(* Logix 5000 AddOnInstructionDefinition export YAI_Assy_72_73_115_EIP_Hz; software revision 21.03 *)

ADD_ON_INSTRUCTION YAI_Assy_72_73_115_EIP_Hz   (* revision 1.0, vendor Yaskawa America, Inc. *)
// YAI Assembly 72/73 and 115
// Help:
// This add-on instruction is for use with input assemblie 72/73 and output assemblies 115.
// Node_Input_Assy is defined as the node's input assembly integer array.
// Node_Output_Assy is defined as the node's output assembly integer array.
// Torque limit/reference, torque compensation and torque output variables are only available with A1000.
VAR_IN_OUT
   Node_Input_Assy : AB:ETHERNET_MODULE_INT_6Bytes:I:0; {required}   // Input assembly words
   Node_Output_Assy : AB:ETHERNET_MODULE_INT_40Bytes:O:0; {required}   // Output assembly words
END_VAR
VAR_INPUT
   RunFwd : BOOL; {visible}   // Forward run command
   RunRev : BOOL; {visible}   // Reverse run command
   MFI_3 : BOOL; {visible}   // Multi-function input 3
   MFI_4 : BOOL; {visible}   // Multi-function input 4
   MFI_5 : BOOL; {visible}   // Multi-function input 5
   MFI_6 : BOOL; {visible}   // Multi-function input 6
   MFI_7 : BOOL; {visible}   // Multi-function input 7
   MFI_8 : BOOL; {visible}   // Multi-function input 8
   External_Fault : BOOL;   // External fault command (EF0)
   FaultReset : BOOL; {visible}   // Fault reset command
   MFO_1 : BOOL; {visible}   // Multi-function output (M1-M2 for A/P1000, MA/MB/MC for V1000)
   MFO_2 : BOOL; {visible}   // Multi-function output (M3-M4 for A/P1000, P1 for V1000)
   MFO_3 : BOOL; {visible}   // Multi-function output (M5-M6 for A/P1000, P2 for V1000)
   Freq_Ref : REAL; {visible}   // Frequency reference command in Hz (xx.xx resolution)
   Torq_Ref_Limit : REAL; {visible}   // Torque reference/limit (A1000 only)
   Torq_Comp : REAL; {visible}   // Torque compensation command (A1000 only)
   Analog_Output_1 : REAL;   // Analog output 1 level command
   Analog_Output_2 : REAL;   // Analog output 2 level command
   Digital_Output_1 : BOOL;   // Digital output 1 activation - M1-M2
   Digital_Output_2 : BOOL;   // Digital output 2 activation - M3-M4
   Digital_Output_3 : BOOL;   // Digital output 3 activation - M5-M6
   Digital_Output_Fault_Enable : BOOL;   // Bit to enable control of fault output relay over the network
   Digital_Output_Fault : BOOL;   // Fault relay activation - MA-MB-MC
END_VAR
VAR_OUTPUT
   At_Speed : BOOL; {access Read Only, visible}   // Drive at commanded speed status bit
   Drive_State : INT; {access Read Only}   // Drive Status - Refer to class 0x29, Instance 0x1, Attribute 0x6 for details
   Faulted : BOOL; {access Read Only, visible}   // Drive faulted status bit
   NetCtrlStatus : BOOL; {access Read Only, visible}   // Drive network run source status bit (1 = source coming from network)
   NetRefStatus : BOOL; {access Read Only, visible}   // Drive network reference status bit (1 = reference coming from network)
   Output_Freq : REAL; {access Read Only, visible}   // Drive output frequency in Hz (xx.xx resolution)
   Ready : BOOL; {access Read Only, visible}   // Drive ready status bit
   RunningFwd : BOOL; {access Read Only, visible}   // Drive running forward status bit
   RunningRev : BOOL; {access Read Only, visible}   // Drive running reverse status bit
   Torque_Actual : REAL; {access Read Only, visible}   // Drive torque output in engineering units.
   Warning : BOOL; {access Read Only, visible}   // Drive warning (alarm) status bit
END_VAR
VAR_INPUT
   Motor_Rated_Torq : REAL := 100.0; {visible}   // Motor rated torque (Engineering units)
END_VAR
VAR
   FRef_Convert : DINT;
   FOut_Convert : REAL;
   FOut_Temp : REAL;
   TRef_Convert : INT;
   TComp_Convert : INT;
   TOut_Convert : REAL;
   TOut_Temp : REAL;
   IOut_Temp : REAL;
   IOut_Convert : REAL;
   AO1_Convert : INT;
   AO2_Convert : INT;
   Motor_Speed_Temp : REAL;
   Motor_Speed_Convert : REAL;
   Freq_Cmd_Temp : REAL;
   Freq_Cmd_Convert : REAL;
   AI1_Temp : REAL;
   AI1_Convert : REAL;
   AI2_Temp : REAL; {access None}
   AI2_Convert : REAL; {access None}
   AI3_Temp : REAL; {access None}
   AI3_Convert : REAL; {access None}
   TOut_Convert1 : REAL;
   Tout_Convert_Temp : REAL;
   TOut_Temp1 : REAL;
   TRef_Convert1 : INT;
   DriveStatusTempBits : INT;
END_VAR

ROUTINE Logic   (* ladder *)
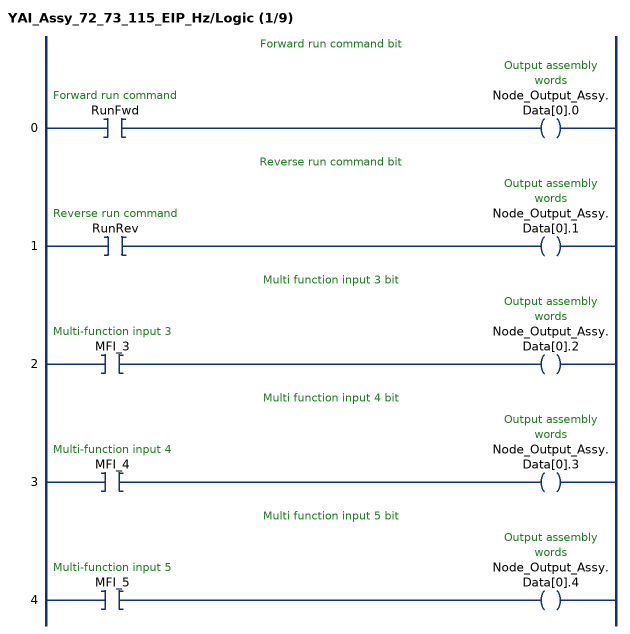
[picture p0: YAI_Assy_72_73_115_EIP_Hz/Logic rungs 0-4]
   // Forward run command bit
   0: XIC(RunFwd)OTE(Node_Output_Assy.Data[0].0);
   // Reverse run command bit
   1: XIC(RunRev)OTE(Node_Output_Assy.Data[0].1);
   // Multi function input 3 bit
   2: XIC(MFI_3)OTE(Node_Output_Assy.Data[0].2);
   // Multi function input 4 bit
   3: XIC(MFI_4)OTE(Node_Output_Assy.Data[0].3);
   // Multi function input 5 bit
   4: XIC(MFI_5)OTE(Node_Output_Assy.Data[0].4);
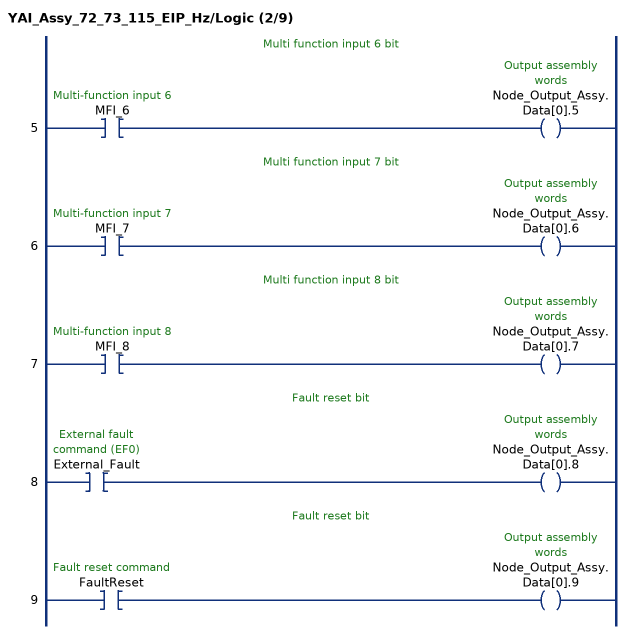
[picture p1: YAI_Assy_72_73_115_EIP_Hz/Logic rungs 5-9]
   // Multi function input 6 bit
   5: XIC(MFI_6)OTE(Node_Output_Assy.Data[0].5);
   // Multi function input 7 bit
   6: XIC(MFI_7)OTE(Node_Output_Assy.Data[0].6);
   // Multi function input 8 bit
   7: XIC(MFI_8)OTE(Node_Output_Assy.Data[0].7);
   // Fault reset bit
   8: XIC(External_Fault)OTE(Node_Output_Assy.Data[0].8);
   // Fault reset bit
   9: XIC(FaultReset)OTE(Node_Output_Assy.Data[0].9);
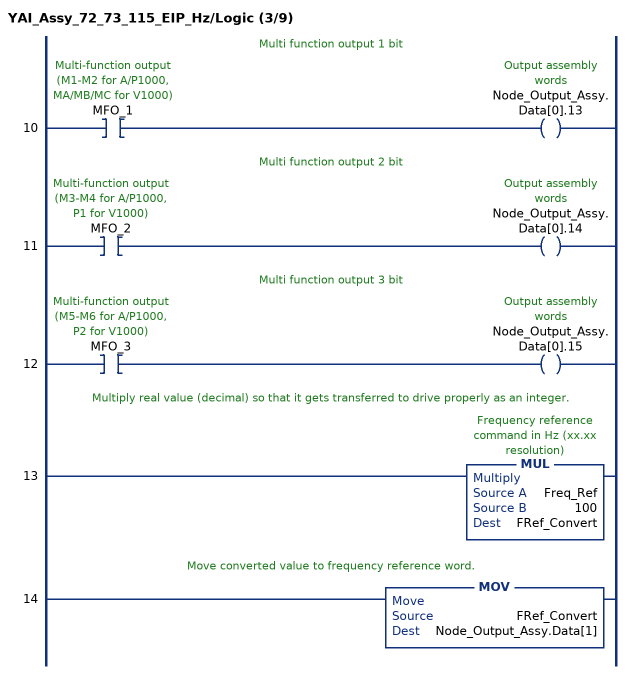
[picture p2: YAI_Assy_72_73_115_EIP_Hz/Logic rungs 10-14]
   // Multi function output 1 bit
   10: XIC(MFO_1)OTE(Node_Output_Assy.Data[0].13);
   // Multi function output 2 bit
   11: XIC(MFO_2)OTE(Node_Output_Assy.Data[0].14);
   // Multi function output 3 bit
   12: XIC(MFO_3)OTE(Node_Output_Assy.Data[0].15);
   // Multiply real value (decimal) so that it gets transferred to drive properly as an integer.
   13: MUL(Freq_Ref,100,FRef_Convert);
   // Move converted value to frequency reference word.
   14: MOV(FRef_Convert,Node_Output_Assy.Data[1]);
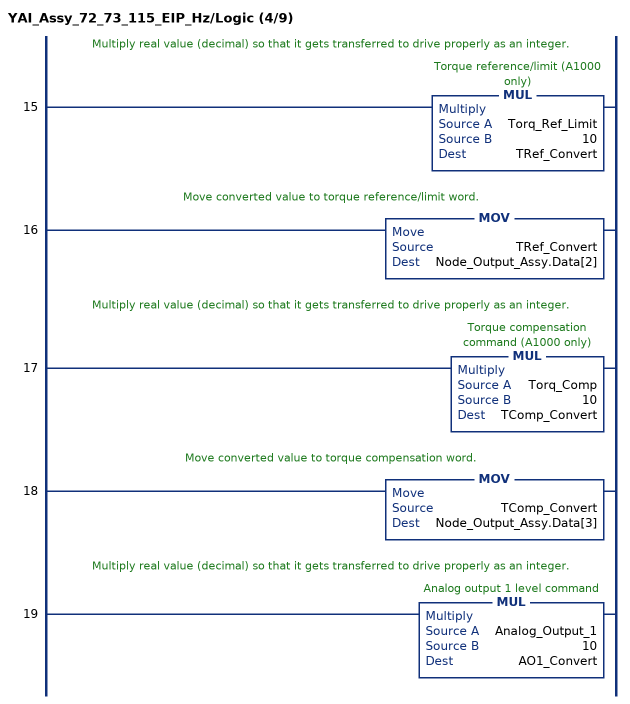
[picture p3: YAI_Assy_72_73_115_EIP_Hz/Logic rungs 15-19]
   // Multiply real value (decimal) so that it gets transferred to drive properly as an integer.
   15: MUL(Torq_Ref_Limit,10,TRef_Convert);
   // Move converted value to torque reference/limit word.
   16: MOV(TRef_Convert,Node_Output_Assy.Data[2]);
   // Multiply real value (decimal) so that it gets transferred to drive properly as an integer.
   17: MUL(Torq_Comp,10,TComp_Convert);
   // Move converted value to torque compensation word.
   18: MOV(TComp_Convert,Node_Output_Assy.Data[3]);
   // Multiply real value (decimal) so that it gets transferred to drive properly as an integer.
   19: MUL(Analog_Output_1,10,AO1_Convert);
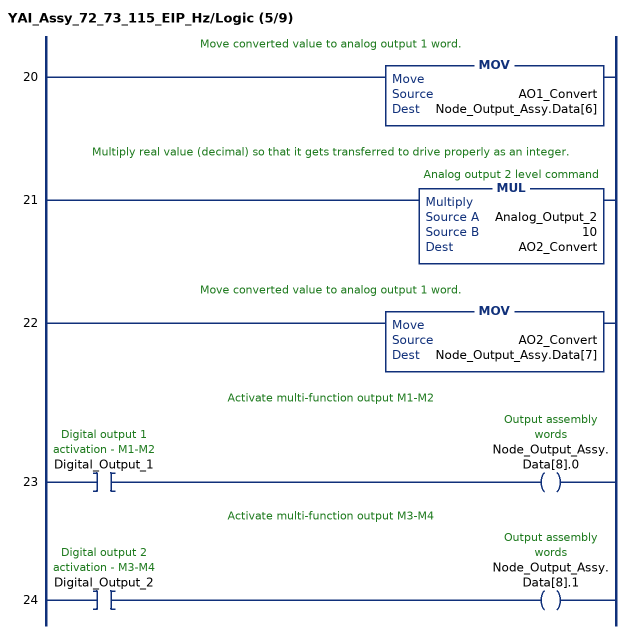
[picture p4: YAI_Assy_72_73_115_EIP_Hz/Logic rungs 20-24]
   // Move converted value to analog output 1 word.
   20: MOV(AO1_Convert,Node_Output_Assy.Data[6]);
   // Multiply real value (decimal) so that it gets transferred to drive properly as an integer.
   21: MUL(Analog_Output_2,10,AO2_Convert);
   // Move converted value to analog output 1 word.
   22: MOV(AO2_Convert,Node_Output_Assy.Data[7]);
   // Activate multi-function output M1-M2
   23: XIC(Digital_Output_1)OTE(Node_Output_Assy.Data[8].0);
   // Activate multi-function output M3-M4
   24: XIC(Digital_Output_2)OTE(Node_Output_Assy.Data[8].1);
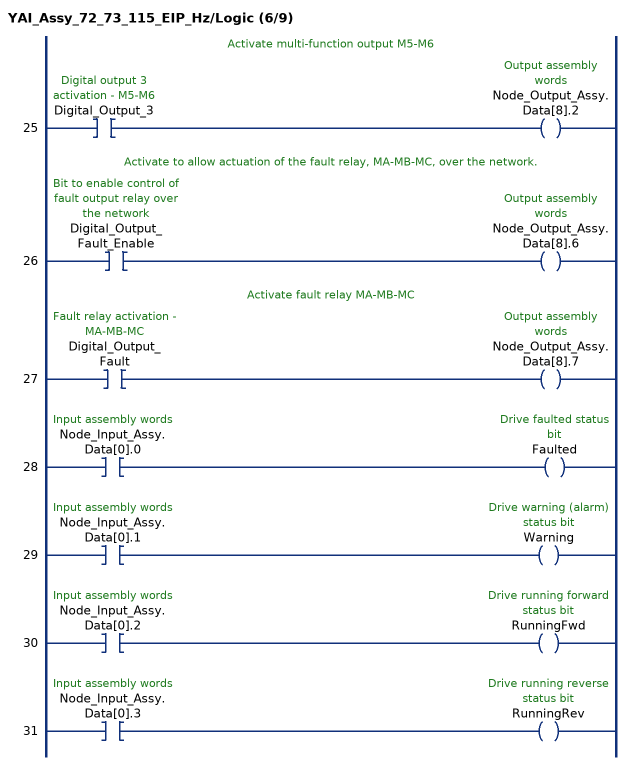
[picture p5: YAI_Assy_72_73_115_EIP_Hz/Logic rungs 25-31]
   // Activate multi-function output M5-M6
   25: XIC(Digital_Output_3)OTE(Node_Output_Assy.Data[8].2);
   // Activate to allow actuation of the fault relay, MA-MB-MC, over the network.
   26: XIC(Digital_Output_Fault_Enable)OTE(Node_Output_Assy.Data[8].6);
   // Activate fault relay MA-MB-MC
   27: XIC(Digital_Output_Fault)OTE(Node_Output_Assy.Data[8].7);
   28: XIC(Node_Input_Assy.Data[0].0)OTE(Faulted);
   29: XIC(Node_Input_Assy.Data[0].1)OTE(Warning);
   30: XIC(Node_Input_Assy.Data[0].2)OTE(RunningFwd);
   31: XIC(Node_Input_Assy.Data[0].3)OTE(RunningRev);
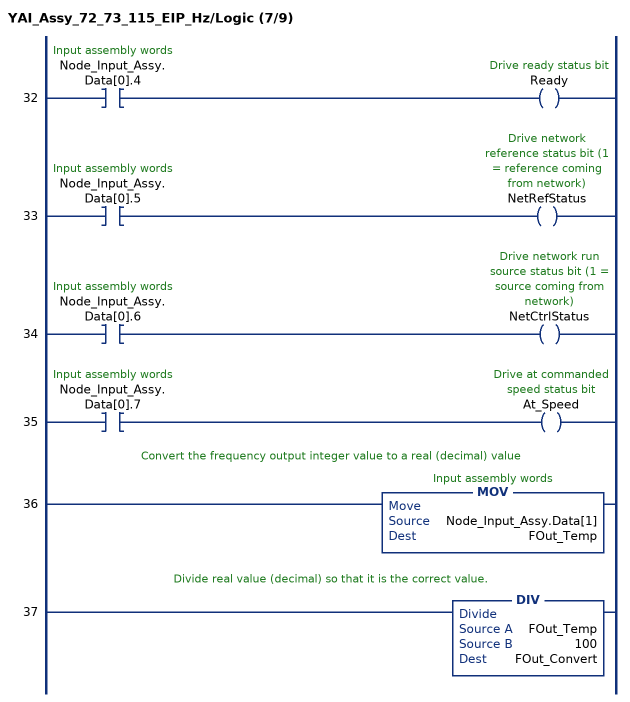
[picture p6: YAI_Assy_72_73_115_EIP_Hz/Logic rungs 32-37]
   32: XIC(Node_Input_Assy.Data[0].4)OTE(Ready);
   33: XIC(Node_Input_Assy.Data[0].5)OTE(NetRefStatus);
   34: XIC(Node_Input_Assy.Data[0].6)OTE(NetCtrlStatus);
   35: XIC(Node_Input_Assy.Data[0].7)OTE(At_Speed);
   // Convert the frequency output integer value to a real (decimal) value
   36: MOV(Node_Input_Assy.Data[1],FOut_Temp);
   // Divide real value (decimal) so that it is the correct value.
   37: DIV(FOut_Temp,100,FOut_Convert);
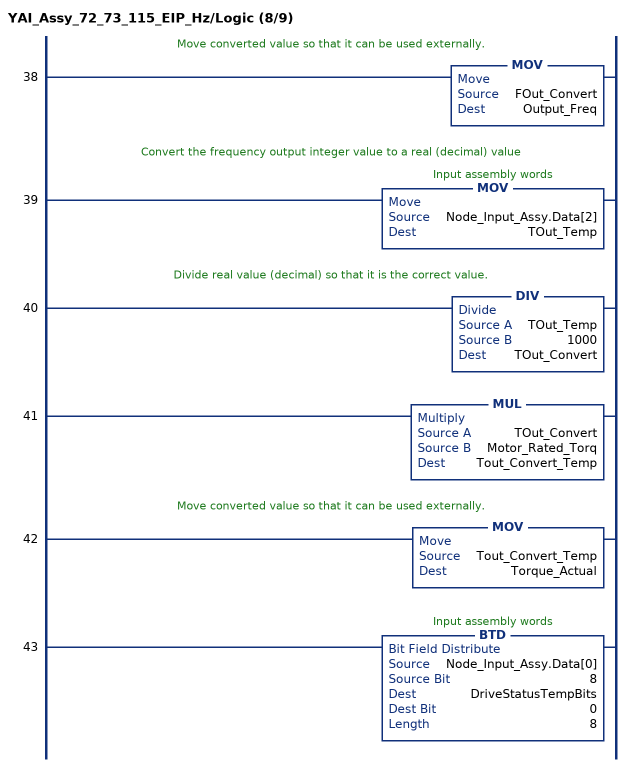
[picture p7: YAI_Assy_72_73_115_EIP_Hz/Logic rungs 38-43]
   // Move converted value so that it can be used externally.
   38: MOV(FOut_Convert,Output_Freq);
   // Convert the frequency output integer value to a real (decimal) value
   39: MOV(Node_Input_Assy.Data[2],TOut_Temp);
   // Divide real value (decimal) so that it is the correct value.
   40: DIV(TOut_Temp,1000,TOut_Convert);
   41: MUL(TOut_Convert,Motor_Rated_Torq,Tout_Convert_Temp);
   // Move converted value so that it can be used externally.
   42: MOV(Tout_Convert_Temp,Torque_Actual);
   43: BTD(Node_Input_Assy.Data[0],8,DriveStatusTempBits,0,8);
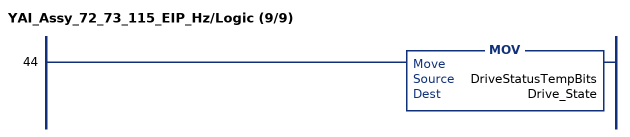
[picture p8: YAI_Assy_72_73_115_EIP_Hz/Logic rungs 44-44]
   44: MOV(DriveStatusTempBits,Drive_State);
END_ROUTINE
END_ADD_ON_INSTRUCTION
